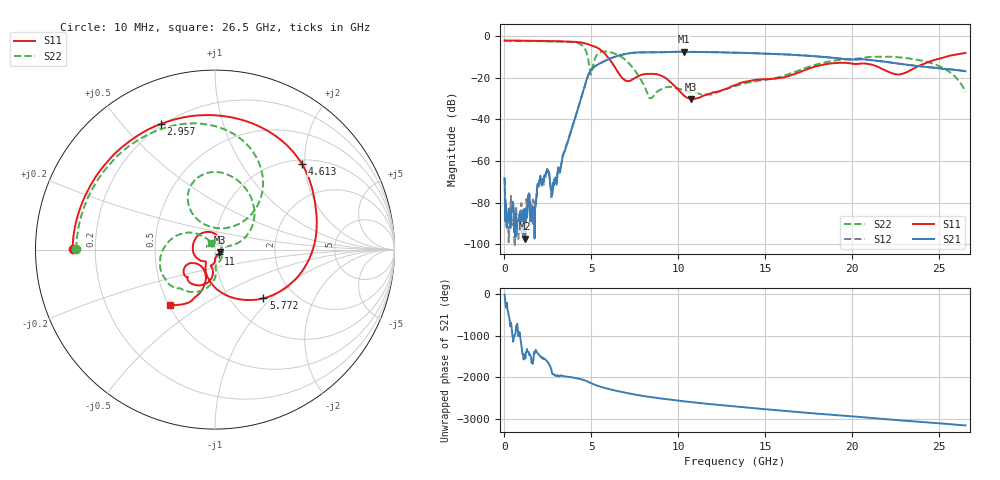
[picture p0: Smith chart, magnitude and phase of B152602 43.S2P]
!  2-Port S-parameters saved by WinCal
! VAR MeasName=S-Parameters (CALIBRATED_DATA) read from VNA (N5242A)
! VAR MeasDate=2016-1-5 16:32:20
! VAR NAME=B152602 43
! VAR FILENAME=B152602 43.S2P
! VAR DATE=2016-1-5 16:32:20
! VAR PHYS_PORTS=1,2
# Hz S DB R 50
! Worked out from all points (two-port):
!   801 points, 10 MHz to 26.5 GHz, reference 50 ohm
!   highest |S21| = -7.43 dB at 10.31 GHz (marker M1); lowest = -97.3 dB at 1.202 GHz (marker M2)
!   |S21| within 3 dB of the highest: 6.157 GHz to 18.96 GHz (12.8 GHz wide, 102 % of centre)
!   lowest |S11| = -30.3 dB at 10.74 GHz (marker M3), VSWR 1.06, Z = 52.7 - j1.63 ohm
!   |S11| at or under -10 dB: 5.943 GHz to 25.32 GHz (19.38 GHz wide, 124 % of centre)
!   |S22| runs from -29.9 to -2.2 dB; largest |S21 - S12| = 0.0026
!   S11 on the Smith chart (normalised r, x): 10 MHz: 0.12, +0.00; 2.957 GHz: 0.19, +0.64; 4.613 GHz: 1.08, +1.93; 5.772 GHz: 1.41, -0.89; 11 GHz: 1.04, -0.05; 26.5 GHz: 0.51, -0.37
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1e7  -2.01 179.7  -68.28 -7.6  -68.01 -91.6  -2.24 179.8
2.08675e8  -2.02 175.7  -86.49 -45.4  -84.91 -133.7  -2.24 176.8
1.20205e9  -2.14 155.3  -97.28 -105.8  -90.08 159.7  -2.31 161.4
1.73185e9  -2.20 143.9  -97.20 16.4  -79.88 85.8  -2.36 152.8
2.427212e9  -2.29 127.7  -64.99 -161.4  -65.87 -162.4  -2.44 140.6
2.957012e9  -2.36 113.4  -68.60 -169.3  -68.36 -169.5  -2.51 129.7
4.447075e9  -3.05 54.4  -28.61 108.4  -28.62 108.5  -4.18 74.1
4.612638e9  -3.34 44.7  -23.88 86.7  -23.90 86.8  -5.76 59.9
4.976875e9  -4.34 22.2  -16.24 17.0  -16.24 17.2  -18.42 84.4
5.771575e9  -8.35 -45.2  -11.82 -98.0  -11.80 -97.9  -7.29 89.5
6.831175e9  -20.53 -123.1  -8.73 157.7  -8.71 157.8  -10.53 42.3
8.35435e9  -18.02 165.0  -7.72 44.9  -7.73 44.8  -29.72 44.1
8.851038e9  -18.46 132.2  -7.71 16.1  -7.70 16.0  -26.22 84.0
1.030799e10  -28.43 15.7  -7.43 -59.0  -7.45 -59.0  -25.94 57.6
1.073845e10  -30.26 -30.2  -7.49 -79.2  -7.48 -79.2  -26.91 49.2
1.100335e10  -29.85 -51.5  -7.52 -91.5  -7.52 -91.4  -27.13 38.0
1.3255e10  -23.46 -90.7  -7.89 175.3  -7.88 175.3  -23.96 -59.3
1.540731e10  -20.42 -103.7  -8.49 94.4  -8.45 94.5  -20.42 -88.4
1.769208e10  -14.99 -100.2  -9.49 12.7  -9.46 12.8  -14.19 -96.7
2.209604e10  -17.18 -146.9  -12.52 -137.2  -12.48 -137.4  -9.83 -159.4
2.507616e10  -10.61 -113.3  -15.50 127.1  -15.46 126.8  -14.64 149.6
2.65e10  -8.03 -129.1  -16.80 78.5  -16.77 78.2  -26.80 122.1
